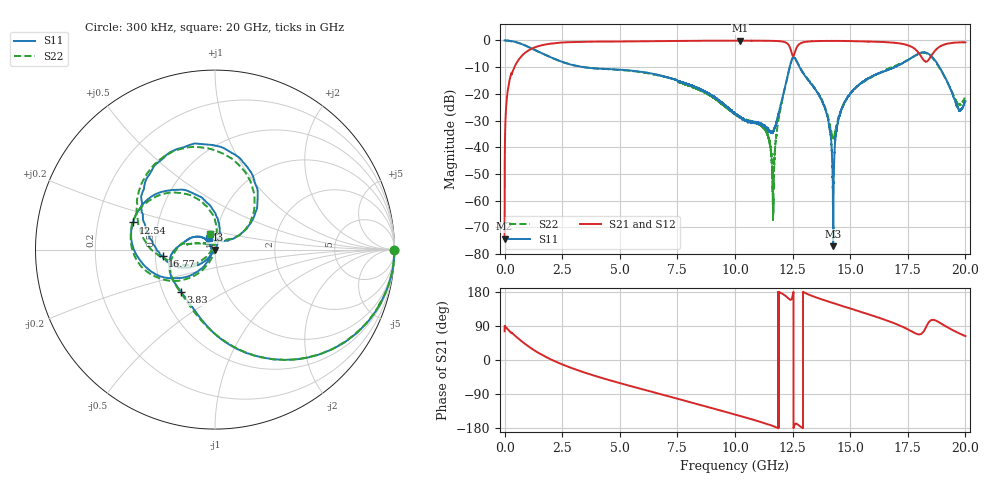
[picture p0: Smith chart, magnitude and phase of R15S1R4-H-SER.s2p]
!{R15S1R4}
!Johanson Technology Inc.
!www.johansontechnology.com
!Test Board Conditions:
!Substrate Type  RO4350B
!Substrate Thickness  20 mil
!Substrate Dk  3.66
!TL Type: GCPW
!TL Trace Width  34 mil
!TL Gap  10 mil
!Electrode orientation  Horizontal
!DUT TOPOLOGY	SERIES
!Mounting Pad LxW  26x52 mil
! Created Sat Feb  6 12:14:04 2021
# hz S ma R 50
! 2 Port Network Data from SP1.SP block
! freq  magS11  angS11  magS21  angS21  magS12  angS12  magS22  angS22
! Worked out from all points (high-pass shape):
!   20001 points, 300 kHz to 20 GHz, reference 50 ohm
!   highest |S21| = -0.07 dB at 10.22 GHz (marker M1); lowest = -74.2 dB at 300 kHz (marker M2)
!   |S21| within 3 dB of the highest: 1.184 GHz to 12.4 GHz (11.22 GHz wide, 165 % of centre); 12.65 GHz to 17.79 GHz (5.137 GHz wide, 33.7 % of centre)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
!   lowest |S11| = -77.0 dB at 14.26 GHz (marker M3), VSWR 1.00, Z = 50 + j0.00448 ohm
!   |S11| at or under -10 dB: 3.43 GHz to 12.37 GHz (8.942 GHz wide, 113 % of centre); 12.8 GHz to 16.93 GHz (4.123 GHz wide, 27.7 % of centre); 18.88 GHz to end of sweep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
!   |S22| runs from -67.3 to 0.0 dB; largest |S21 - S12| = 0.016
!   S11 on the Smith chart (normalised r, x): 300 kHz: open; 3.83 GHz: 0.62, -0.32; 12.54 GHz: 0.36, +0.14; 16.77 GHz: 0.55, -0.05; 20 GHz: 0.93, +0.12
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300000  1 -0.2  0.000194 75.6  0.0002209 82.5  0.9978 -0.2
1.313e8  0.9934 -8.2  0.1114 81.5  0.112 81.5  0.9923 -8.2
5.043e8  0.9272 -28.3  0.3708 61.4  0.3718 61.6  0.9262 -28.2
1.7823e9  0.5339 -81.5  0.842 8.4  0.8426 8.4  0.5329 -81.5
3.3343e9  0.3207 -119.1  0.9434 -30.3  0.9432 -30.4  0.3225 -120.9
3.8303e9  0.3021 -128.6  0.9491 -40.1  0.9494 -40.1  0.3032 -130.9
6.6673e9  0.2263 -179.5  0.9671 -88.4  0.9685 -88.4  0.2229 -177.5
1.00003e10  0.0424 133.1  0.9901 -144.0  0.9908 -143.9  0.04226 130.0
1.02183e10  0.03725 135.2  0.9922 -147.7  0.9902 -147.6  0.03699 121.5
1.13063e10  0.02496 152.3  0.9844 -167.2  0.9863 -167.2  0.02207 79.7
1.16513e10  0.01976 -165.1  0.9814 -174.2  0.9804 -174.2  0.0004334 -34.0
1.19443e10  0.05307 -123.3  0.9684 178.3  0.9689 178.4  0.04534 -109.9
1.25363e10  0.4809 161.6  0.5115 179.0  0.515 178.3  0.4824 166.6
1.33343e10  0.1487 81.1  0.9649 169.3  0.9644 169.4  0.1506 88.9
1.39643e10  0.0437 66.9  0.979 156.1  0.9784 156.0  0.04638 87.5
1.42603e10  0.0001411 161.5  0.9813 150.2  0.9801 150.2  0.01528 151.4
1.44743e10  0.03081 -125.1  0.9805 146.0  0.9788 146.0  0.03404 -148.6
1.48233e10  0.07726 -130.9  0.9769 139.2  0.9776 139.4  0.07799 -140.5
1.66673e10  0.2832 -169.6  0.9242 102.5  0.9115 102.5  0.2968 -171.4
1.67663e10  0.2938 -172.6  0.9194 100.4  0.9041 100.3  0.3094 -173.1
1.83273e10  0.5831 91.4  0.4049 91.2  0.4047 91.7  0.5697 96.0
2e10  0.07258 118.7  0.9221 63.0  0.9185 62.9  0.09096 108.7
